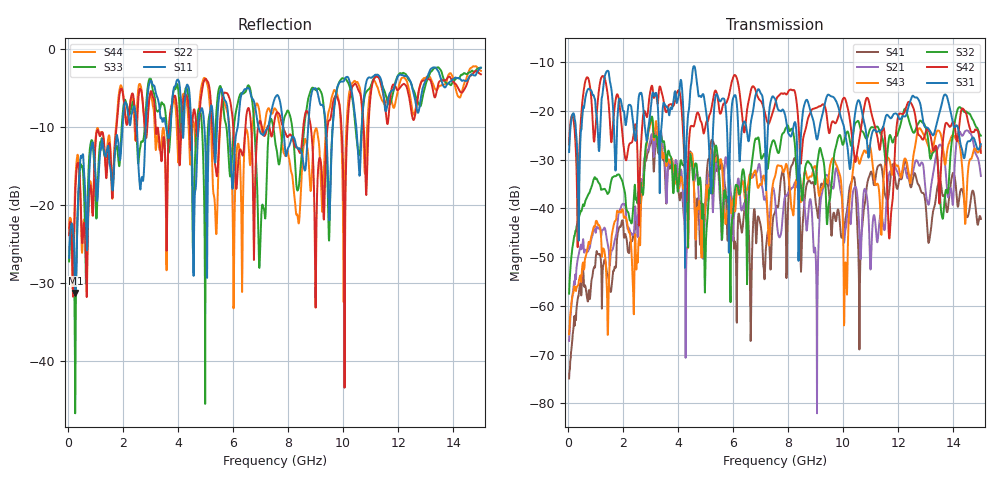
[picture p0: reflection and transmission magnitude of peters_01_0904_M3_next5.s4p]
# MHZ S RI R 50.00
! FREQ  S11  S12  S13  S14
!  S21  S22  S23  S24
!  S31  S32  S33  S34
!  S41  S42  S43  S44
!  REAL  IMAG  REAL  IMAG  REAL  IMAG  REAL  IMAG
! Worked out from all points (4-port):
!   1496 points, 50 MHz to 15 GHz, reference 50 ohm
!   strongest paths, dB at 50 MHz, 3.79 GHz, 7.53 GHz, 11.27 GHz, 15 GHz:
!     S31: -28.5, -19.6, -17.6, -24.2, -26.9
!     S42: -26.9, -19.0, -18.6, -26.3, -28.6
!     S32: -57.5, -32.1, -26.7, -23.4, -25.1
!     S43: -65.8, -30.0, -33.4, -35.2, -27.3
!     S21: -67.2, -30.8, -38.3, -45.7, -33.4
!     S41: -74.9, -30.2, -40.7, -31.3, -42.2
!   lowest |S11| = -31.3 dB at 280 MHz (marker M1), VSWR 1.06, Z = 47.4 + j0.15 ohm
!   |S11| at or under -10 dB: start of sweep to 1.987 GHz; 6.922 GHz to 7.28 GHz (358.5 MHz wide, 5.05 % of centre); 7.824 GHz to 8.729 GHz (905 MHz wide, 10.9 % of centre)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
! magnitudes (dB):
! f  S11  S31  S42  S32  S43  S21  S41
! 50 MHz  -26.8  -28.5  -26.9  -57.5  -65.8  -67.2  -74.9
! 280 MHz  -31.3  -22.5  -26.5  -44.6  -56.1  -53.5  -62.0
! 3.02 GHz  -4.1  -19.1  -15.4  -21.7  -22.3  -25.3  -26.2
! 5.01 GHz  -14.3  -19.7  -22.9  -48.2  -38.6  -39.8  -37.4
! 9.65 GHz  -8.5  -17.2  -22.2  -30.3  -29.8  -35.8  -41.0
! 10.09 GHz  -3.7  -25.3  -17.8  -25.0  -51.1  -44.1  -42.0
! 15 GHz  -2.4  -26.9  -28.6  -25.1  -27.3  -33.4  -42.2
